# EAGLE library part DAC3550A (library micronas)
MPEG3 DECODER update 14.05.2001 librarian@cadsoft.de
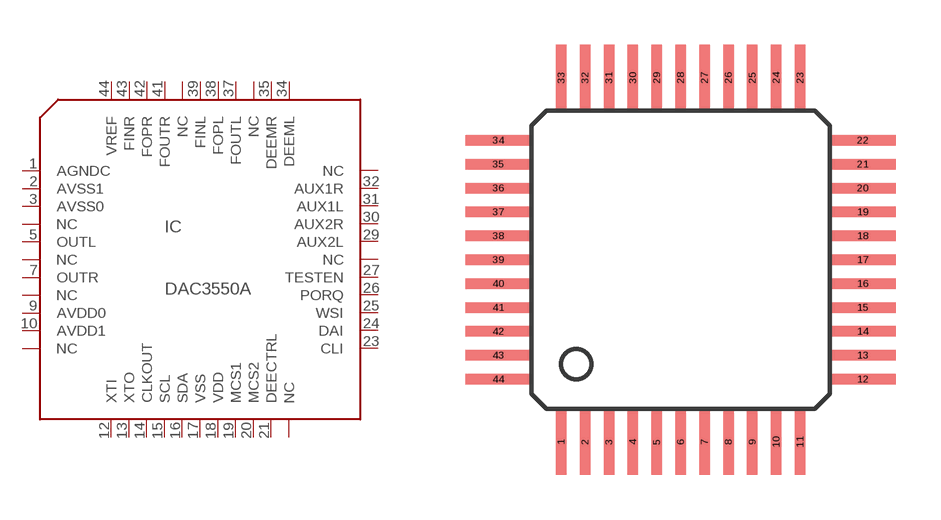
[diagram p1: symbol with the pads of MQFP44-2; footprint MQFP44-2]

Designator prefix IC

## DAC3550AD (OC_FARNELL: unknown; OC_NEWARK: unknown)  [MQFP44-2]
1  AGNDC
2  AVSS1  in
3  AVSS0  in
4  NC4  nc
5  OUTL  out
6  NC6  nc
7  OUTR  out
8  NC8  nc
9  AVDD0  in
10  AVDD1  in
11  NC11  nc
12  XTI  in
13  XTO
14  CLKOUT  out
15  SCL
16  SDA
17  VSS  pwr
18  VDD  pwr
19  MCS1  in
20  MCS2  in
21  DEECTRL  in
22  NC22  nc
23  CLI  in
24  DAI  in
25  WSI  in
26  PORQ  in
27  TESTEN  in
28  NC28  nc
29  AUX2L  in
30  AUX2R  in
31  AUX1L  in
32  AUX1R  in
33  NC33  nc
34  DEEML  out
35  DEEMR  out
36  NC36  nc
37  FOUTL  out
38  FOPL
39  FINL
40  NC40  nc
41  FOUTR  out
42  FOPR
43  FINR
44  VREF  in

## Footprint MQFP44-2 (pad centres in mm)
Metric Quad Flat Pack
smd 0.35 x 2.2: 1 -4,-6.1; 2 -3.2,-6.1; 3 -2.4,-6.1; 4 -1.6,-6.1; 5 -0.8,-6.1; 6 0,-6.1; 7 0.8,-6.1; 8 1.6,-6.1; 9 2.4,-6.1; 10 3.2,-6.1; 11 4,-6.1; 23 4,6.1; 24 3.2,6.1; 25 2.4,6.1; 26 1.6,6.1; 27 0.8,6.1; 28 0,6.1; 29 -0.8,6.1; 30 -1.6,6.1; 31 -2.4,6.1; 32 -3.2,6.1; 33 -4,6.1
smd 2.2 x 0.35: 12 6.1,-4; 13 6.1,-3.2; 14 6.1,-2.4; 15 6.1,-1.6; 16 6.1,-0.8; 17 6.1,0; 18 6.1,0.8; 19 6.1,1.6; 20 6.1,2.4; 21 6.1,3.2; 22 6.1,4; 34 -6.1,4; 35 -6.1,3.2; 36 -6.1,2.4; 37 -6.1,1.6; 38 -6.1,0.8; 39 -6.1,0; 40 -6.1,-0.8; 41 -6.1,-1.6; 42 -6.1,-2.4; 43 -6.1,-3.2; 44 -6.1,-4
